TYPE LstHeater :
STRUCT
	ToleranceMode:STRING;		//'Value' or 'Percent'
	ToleranceDelayTime:INT;
	WallTemp:INT;
	WallTempWaningRange:INT;
	WallTempAlarmRange:INT;
	
	LidTemp:INT;
	LidTempWaningRange:INT;
	LidTempAlarmRange:INT;
	
	StageTemp1: INT;
	StageTemp1WaningRange:INT;
	StageTemp1AlarmRange:INT;
	
	StageTemp2: INT;
	StageTemp2WaningRange:INT;
	StageTemp2AlarmRange:INT;
	
	StageTemp3: INT;
	StageTemp3WaningRange:INT;
	StageTemp3AlarmRange:INT;
	
	StageTemp4: INT;
	StageTemp4WaningRange:INT;
	StageTemp4AlarmRange:INT;
	
END_STRUCT
END_TYPE
